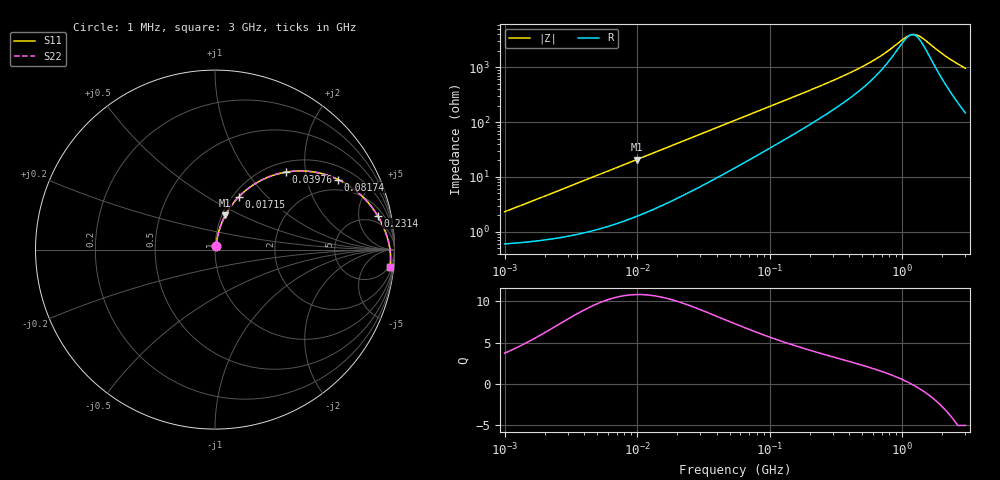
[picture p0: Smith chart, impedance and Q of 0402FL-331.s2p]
# MHz S MA R 50
!Freq  MagS11  AngS11  MagS21  AngS21  MagS12  AngS12  MagS22  AngS22
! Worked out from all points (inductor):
!   801 points, 1 MHz to 3 GHz, reference 50 ohm
!   read as one part in series: L = 353 nH near 1.041 MHz
!   highest Q = 10.8 at 9.893 MHz (marker M1), where L = 331 nH
!   self-resonance near 1.177 GHz
!   S11 on the Smith chart (normalised r, x): 1 MHz: 1.01, +0.04; 17.15 MHz: 1.07, +0.70; 39.76 MHz: 1.19, +1.57; 81.74 MHz: 1.50, +3.12; 231.4 MHz: 3.23, +8.47; 3 GHz: 4, -19
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1  0.02302 73.8  0.9938 -1.3  0.9938 -1.3  0.02302 73.8
3.823119  0.08153 78.9  0.9875 -4.6  0.9875 -4.6  0.08153 78.9
6.242973  0.1297 77.0  0.9791 -7.4  0.9791 -7.4  0.1297 77.0
9.892953  0.1986 73.3  0.962 -11.4  0.962 -11.4  0.1986 73.3
14.47069  0.2785 68.5  0.9346 -16.1  0.9346 -16.1  0.2785 68.5
17.1545  0.3217 65.8  0.9163 -18.7  0.9163 -18.7  0.3217 65.8
25.85714  0.4435 57.8  0.8506 -26.2  0.8506 -26.2  0.4435 57.8
39.76269  0.586 47.5  0.7425 -35.6  0.7425 -35.6  0.586 47.5
54.77226  0.6869 39.3  0.6394 -42.9  0.6394 -42.9  0.6869 39.3
81.73662  0.79 29.6  0.5 -51.3  0.5 -51.3  0.79 29.6
128.2345  0.8686 20.4  0.3555 -58.5  0.3555 -58.5  0.8686 20.4
209.4008  0.9183 13.0  0.2319 -63.0  0.2319 -63.0  0.9183 13.0
231.4421  0.9252 11.8  0.2112 -63.5  0.2112 -63.5  0.9252 11.8
480.5402  0.9577 5.2  0.09804 -61.9  0.09804 -61.9  0.9577 5.2
629.6259  0.9646 3.4  0.06867 -57.3  0.06867 -57.3  0.9646 3.4
792.5923  0.9693 2.1  0.04753 -48.7  0.04753 -48.7  0.9693 2.1
1091.779  0.9743 0.4  0.02662 -14.7  0.02662 -14.7  0.9743 0.4
1182.785  0.9753 -0.0  0.02472 1.0  0.02472 1.0  0.9753 -0.0
1268.618  0.9761 -0.4  0.02486 15.7  0.02486 15.7  0.9761 -0.4
1430.499  0.9773 -1.0  0.0289 37.8  0.0289 37.8  0.9773 -1.0
2221.924  0.9799 -3.6  0.06586 70.4  0.06586 70.4  0.9799 -3.6
3000  0.9793 -5.8  0.102 75.4  0.102 75.4  0.9793 -5.8
